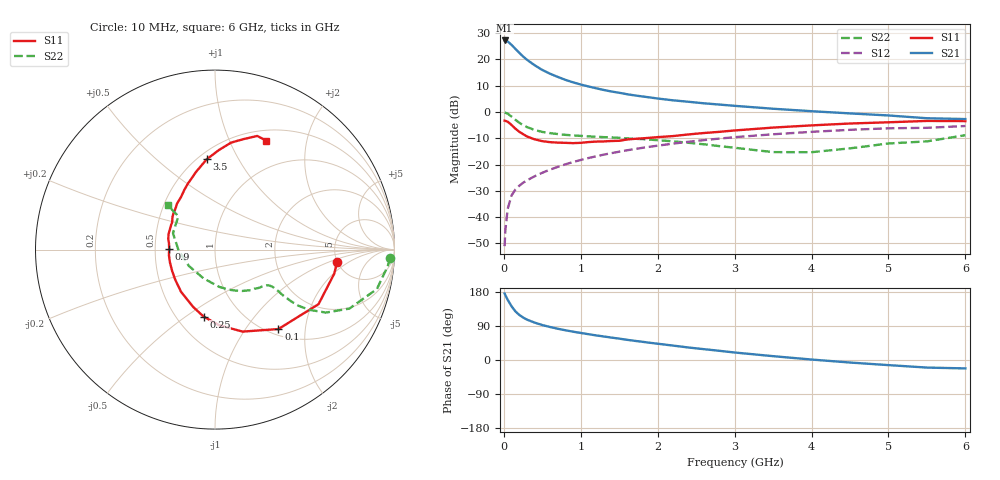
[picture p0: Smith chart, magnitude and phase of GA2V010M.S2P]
! Infineon Technologies  Discrete & RF Semiconductors
! BF775
! Si NPN RF Bipolar Junction Transistor in SOT23
! VCE = 2 V  IC = 10 mA
! Common Emitter S-Parameters:  May  1996
# GHz  S  MA  R  50
!  f  S11  S21  S12  S22
! GHz  MAG  ANG  MAG  ANG  MAG  ANG  MAG  ANG
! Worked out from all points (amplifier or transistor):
!   36 points, 10 MHz to 6 GHz, reference 50 ohm
!   highest |S21| = 27.2 dB at 10 MHz (marker M1)
!   |S21| within 3 dB of that: start of sweep to 143.8 MHz
!   unconditionally stable (mu >= 1): 528.3 MHz to 3.759 GHz
!   at 250 MHz: K = 0.70, MSG = 24.0 dB, |S12| = -26.9 dB
!   at 1.4 GHz: K = 1.13, MAG = 9.5 dB, |S12| = -15.7 dB
!   at 6 GHz: K = 0.99, MSG = 1.3 dB, |S12| = -5.3 dB
!   S11 on the Smith chart (normalised r, x): 10 MHz: 5.00, -1.28; 100 MHz: 1.11, -1.44; 250 MHz: 0.67, -0.59; 900 MHz: 0.59, +0.01; 3.5 GHz: 0.55, +0.75; 6 GHz: 0.63, +1.38
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0.01  0.6848 -5.7  22.92 175.7  0.0028 87.9  0.9781 -2.7
0.02  0.6775 -11.5  22.87 171.0  0.0057 84.2  0.966 -5.6
0.05  0.6521 -27.8  21.93 158.9  0.0143 78.0  0.9284 -13.7
0.1  0.5663 -51.4  18.92 141.9  0.0258 67.9  0.8177 -23.7
0.15  0.4821 -71.4  15.88 128.3  0.0334 62.8  0.7104 -29.6
0.2  0.4215 -86.9  13.4 119.1  0.0394 61.4  0.625 -32.5
0.25  0.3788 -99.6  11.37 112.1  0.045 60.1  0.5619 -33.9
0.3  0.3425 -110.6  9.86 106.6  0.05 60.5  0.5163 -34.2
0.4  0.3018 -128.8  7.744 98.7  0.0598 61.2  0.4547 -33.9
0.5  0.2782 -142.6  6.295 92.2  0.0697 62.3  0.4172 -33.2
0.6  0.2667 -153.7  5.344 87.1  0.08 62.7  0.3963 -33.0
0.7  0.2611 -164.1  4.647 82.5  0.0901 63.4  0.3802 -32.9
0.9  0.2554 178.8  3.66 74.7  0.1117 63.2  0.3578 -33.7
1.1  0.2674 166.9  3.056 68.1  0.1329 62.6  0.3439 -35.9
1.3  0.2752 156.0  2.619 62.0  0.1544 61.1  0.3321 -38.4
1.6  0.2992 142.3  2.177 53.3  0.1865 58.5  0.3148 -43.4
2.2  0.3479 123.1  1.665 38.0  0.2499 52.4  0.2763 -56.5
2.8  0.4187 108.0  1.384 24.3  0.3115 44.9  0.2243 -75.4
3.5  0.5048 95.3  1.152 10.1  0.3765 35.5  0.1723 -112.0
4.5  0.6031 81.4  0.939 -6.7  0.4576 22.0  0.2032 -178.7
5.5  0.6756 69.6  0.76 -20.0  0.4995 7.6  0.2758 137.7
6  0.6709 64.7  0.733 -22.2  0.5405 3.6  0.3615 136.8
